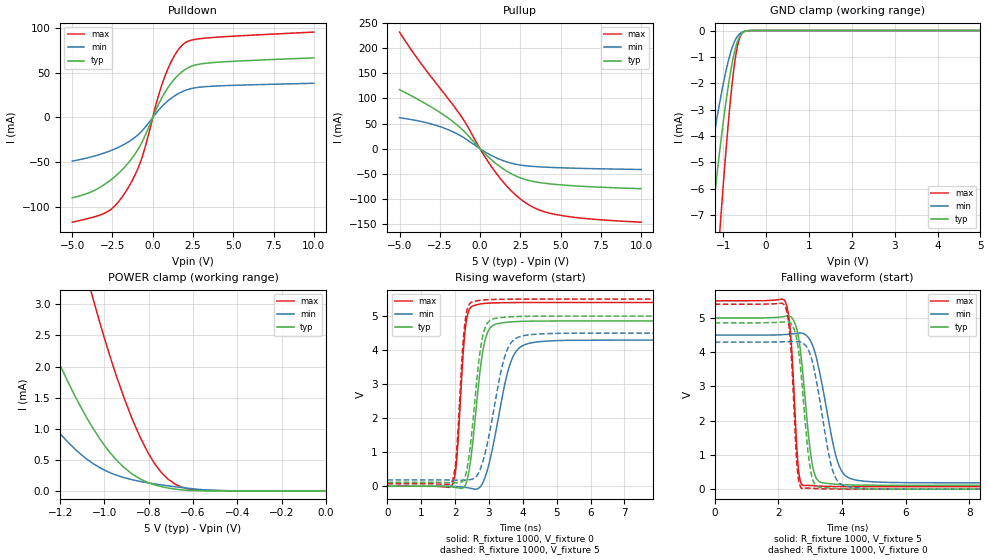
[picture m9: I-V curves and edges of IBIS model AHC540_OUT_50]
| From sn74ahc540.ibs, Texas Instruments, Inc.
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[Model]   AHC540_OUT_50
Model_type  3-state
Enable   Active-Low
Vref =   0
Rref =   1000
Cref =   50p
Vmeas =   2.5
| variable   typ   min   max
C_comp   2.46pF   2.27pF   2.54pF
| C_pullup   3.48pF   2.52pF   4.35pF
| C_pulldown   3.03pF   2.60pF   3.75pF
| C_tri-state   2.46pF   2.27pF   2.54pF
[Temperature Range]   40   100   -40
| Ambient temperature   25   85   -40
[Voltage range]   5   4.5   5.5
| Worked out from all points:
|   slope of the pulldown table from 0 to 0.75 V, typ, clamps not added: 27.1 ohm
|   slope of the pullup table from 0 to 0.75 V, typ, clamps not added: 32.2 ohm
|   GND clamp passes 1 mA (typ) near -0.76 V on its own axis
|   POWER clamp passes 1 mA (typ) near -1.05 V on its own axis
|   rising waveform, R_fixture 1000, V_fixture 0: 20-80 % time 320ps typ, 526ps min, 201ps max; typ from 0 V to 4.86 V
|   falling waveform, R_fixture 1000, V_fixture 5: 20-80 % time 311ps typ, 542ps min, 189ps max; typ from 5 V to 0.113 V
|   rising waveform, R_fixture 1000, V_fixture 5: 20-80 % time 309ps typ, 514ps min, 197ps max; typ from 0.113 V to 5 V
|   falling waveform, R_fixture 1000, V_fixture 0: 20-80 % time 291ps typ, 482ps min, 182ps max; typ from 4.86 V to 0 V
[GND Clamp]
| AHC540_OUT_50
|   Voltage   I(typ)   I(min)   I(max)
-5V       -95.67mA   -62.49mA   -121.3mA
-1.555V   -12.25mA   -7.735mA   -19.36mA
-1.505V   -11.34mA   -7.146mA   -18.05mA
-1.3V     -7.837mA   -4.868mA   -12.82mA
-1.25V    -7.04mA    -4.349mA   -11.6mA
-1.075V   -4.462mA   -2.668mA   -7.496mA
-1.055V   -4.191mA   -2.491mA   -7.052mA
-895mV    -2.233mA   -1.242mA   -3.755mA
-765mV    -1.017mA   -526.9uA   -1.617mA
-665mV    -407.3uA   -211.2uA   -563.1uA
-545mV    -77.75uA   -49.36uA   -79.99uA
5V        35.47nA    7.112uA    323.5nA
[POWER Clamp]
| AHC540_OUT_50
|   Voltage   I(typ)   I(min)   I(max)
-5V       75.68mA    48.36mA    122.9mA
-1.6V     5.955mA    3.194mA    12.64mA
-1.345V   3.264mA    1.609mA    7.646mA
-1.315V   2.988mA    1.452mA    7.117mA
-1.195V   1.981mA    900.5uA    5.137mA
-1.075V   1.146mA    499uA      3.399mA
-1.05V    997.6uA    437uA      3.071mA
-945mV    493.1uA    251.9uA    1.837mA
-840mV    195.2uA    153.7uA    872.8uA
-715mV    48.24uA    82.85uA    195.1uA
-590mV    4.193uA    30.5uA     16.89uA
-84.45fV  35.47nA    2.067nA    492nA
[Pulldown]
| AHC540_OUT_50
|   Voltage   I(typ)   I(min)   I(max)
-5V       -89.39mA   -48.52mA   -116.5mA
-3.785V   -82.48mA   -43.7mA    -111.4mA
-2.8V     -72.09mA   -38.21mA   -104.7mA
-2.245V   -64.06mA   -34.17mA   -96.27mA
-1.62V    -52.73mA   -28.37mA   -80.95mA
-700mV    -28.6mA    -15.56mA   -46.32mA
310mV     12.8mA     7.047mA    21.54mA
795mV     29.02mA    16.15mA    47.75mA
1.365V    43.04mA    24.14mA    69.33mA
1.925V    52.34mA    29.44mA    82.07mA
3.485V    60.67mA    34.55mA    88.62mA
10V       66.28mA    38.05mA    95mA
[Pullup]
| AHC540_OUT_50
|   Voltage   I(typ)   I(min)   I(max)
-5V       117.7mA    61.62mA    232.2mA
-3.725V   95.86mA    54.62mA    172.4mA
-1.745V   55.47mA    34.54mA    89.9mA
-935mV    32.81mA    20.42mA    53mA
120mV     -4.081mA   -2.548mA   -6.465mA
885mV     -26.97mA   -16.38mA   -43.74mA
1.7V      -45.52mA   -26.69mA   -75.96mA
2.515V    -58.22mA   -32.71mA   -100.4mA
3.525V    -66.57mA   -35.81mA   -120.1mA
4.76V     -71.38mA   -37.74mA   -131.4mA
6.775V    -75.68mA   -39.6mA    -139.7mA
10V       -79.63mA   -41.43mA   -146.4mA
[Ramp]
| AHC540_OUT_50
| variable   typ   min   max
dV/dt_r   2.95/3.28E-10   2.63/5.41E-10   3.26/2.05E-10
dV/dt_f   2.97/3.24E-10   2.63/5.55E-10   3.29/1.95E-10
R_load = 1000
[Rising Waveform]
| AHC540_OUT_50
R_fixture =   1000
C_fixture =   0
L_fixture =   0
V_fixture =   0
V_fixture_min = 0
V_fixture_max = 0
|   Time   V(typ)   V(min)   V(max)
0s        1.739nV    2.898nV    1.09nV
1.91ns    -22.63mV   -3.081mV   23.29mV
2.04ns    -39.93mV   -10.05mV   705.4mV
2.245ns   -36.96mV   -28.6mV    4.006V
2.34ns    140.6mV    -40.83mV   4.905V
2.845ns   4.117V     158.7mV    5.369V
3.065ns   4.686V     929.2mV    5.384V
3.68ns    4.831V     3.741V     5.396V
4.565ns   4.854V     4.255V     5.399V
50ns      4.857V     4.295V     5.4V
[Falling Waveform]
| AHC540_OUT_50
R_fixture =   1000
C_fixture =   0
L_fixture =   0
V_fixture =   5
V_fixture_min = 4.5
V_fixture_max = 5.5
|   Time   V(typ)   V(min)   V(max)
0s        5V         4.5V       5.5V
2.21ns    5.047V     4.516V     5.496V
2.385ns   5.04V      4.529V     4.538V
2.63ns    4.458V     4.558V     602.6mV
2.795ns   3.131V     4.541V     102.6mV
3.02ns    998.2mV    4.314V     106.6mV
3.195ns   312.9mV    3.841V     94.18mV
3.9ns     137.8mV    705.7mV    77.05mV
4.7ns     117.7mV    232.2mV    73.65mV
50ns      112.6mV    184.5mV    72.6mV
[Rising Waveform]
| AHC540_OUT_50
R_fixture =   1000
C_fixture =   0
L_fixture =   0
V_fixture =   5
V_fixture_min = 4.5
V_fixture_max = 5.5
|   Time   V(typ)   V(min)   V(max)
0s        112.6mV    184.5mV    72.6mV
1.91ns    100.7mV    181.9mV    134mV
2.03ns    99.84mV    178.5mV    851.4mV
2.22ns    144.5mV    175.7mV    4.017V
2.32ns    368.4mV    179.3mV    5.018V
2.79ns    4.286V     637.1mV    5.469V
3.015ns   4.862V     1.559V     5.484V
3.525ns   4.971V     3.975V     5.495V
4.32ns    4.996V     4.463V     5.499V
50ns      5V         4.5V       5.5V
[Falling Waveform]
| AHC540_OUT_50
R_fixture =   1000
C_fixture =   0
L_fixture =   0
V_fixture =   0
V_fixture_min = 0
V_fixture_max = 0
|   Time   V(typ)   V(min)   V(max)
0s        4.857V     4.295V     5.4V
2.205ns   4.884V     4.306V     5.368V
2.375ns   4.857V     4.309V     4.347V
2.6ns     4.272V     4.309V     550.3mV
2.735ns   3.15V      4.285V     19.31mV
2.94ns    1.024V     4.069V     31.7mV
3.11ns    205.5mV    3.561V     22.79mV
3.72ns    25.52mV    512.4mV    5.699mV
4.395ns   6.365mV    44.82mV    1.665mV
50ns      -1.938nV   -7.502nV   -599.8pV
